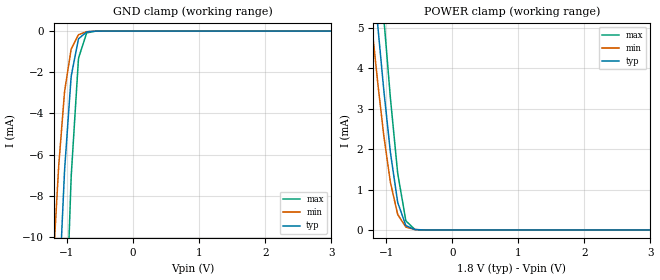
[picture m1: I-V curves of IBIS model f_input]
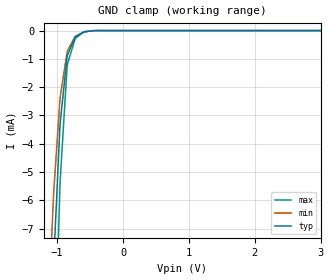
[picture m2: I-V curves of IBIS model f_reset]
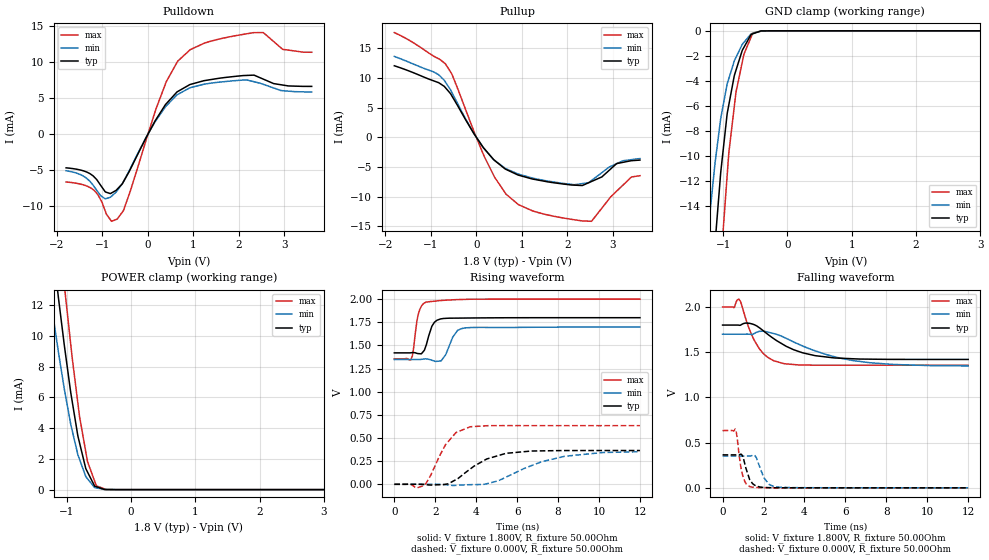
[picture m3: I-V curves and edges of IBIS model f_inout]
[IBIS Ver]   3.2
[File Name]   rc_p30_18v_64m_b.ibs
[File Rev]   1.01
[Date]   3/10/2010
[Source]   From silicon level SPICE model at Numonyx B.V.
[Notes]   The following information corresponds to the 65nm
   Redcliff P30 64Mb chip with EZBGA package.
[Disclaimer]   This information is for modeling purposes only and is not
   guaranteed.Numonyx B.V. is not responsible for any problem
   this model may cause to customers.
[Copyright]   Copyright 2010, Numonyx B.V., All Rights Reserved.
[Component]   P30_18V_64M_EZBGA
[Manufacturer]  Numonyx B.V.
[Package]
|   typ   min   max
R_pkg   0.35Ohm   0.18Ohm   0.51Ohm
L_pkg   7.00nH   3.67nH   10.32nH
C_pkg   1.26pF   0.74pF   1.77pF
[PIN]   signal_name   model_name   R_pin   L_pin   C_pin
A1   A1   f_input   0.29   6.04nH   1.07pF
A2   A6   f_input   0.38   7.66nH   1.33pF
A3   A8   f_input   0.23   4.81nH   0.86pF
A4   NC   NC
A5   A13   f_input   0.23   4.78nH   0.86pF
A6   VCC   POWER
A7   A18   f_input   0.30   6.53nH   1.17pF
A8   A22   f_input   0.35   7.76nH   1.27pF
B1   A2   f_input   0.29   5.78nH   1.02pF
B2   VSS   GND
B3   A9   f_input   0.36   7.42nH   1.29pF
B4   CE#   f_input   0.41   7.76nH   1.27pF
B5   A14   f_input   0.24   4.84nH   0.86pF
B6   NC   NC
B7   A19   f_input   0.29   6.32nH   1.13pF
B8   NC   NC
C1   A3   f_input   0.30   6.01nH   1.05pF
C2   A7   f_input   0.31   6.07nH   1.06pF
C3   A10   f_input   0.35   7.09nH   1.24pF
C4   A12   f_input   0.34   6.90nH   1.20pF
C5   A15   f_input   0.28   5.58nH   0.98pF
C6   WP#   f_input   0.28   5.60nH   0.99pF
C7   A20   f_input   0.43   8.80nH   1.52pF
C8   A21   f_input   0.35   7.07nH   1.24pF
D1   A4   f_input   0.32   6.32nH   1.10pF
D2   A5   f_input   0.30   5.77nH   1.00pF
D3   A11   f_input   0.37   7.56nH   1.31pF
D4   RST#   f_reset   0.35   6.65nH   1.20pF
D5   VCCQ   POWER
D6   VCCQ   POWER
D7   A16   f_input   0.28   5.43nH   0.94pF
D8   A17   f_input   0.30   5.95nH   1.04pF
E1   DQ8   f_inout   0.30   6.55nH   1.21pF
E2   DQ1   f_inout   0.28   5.48nH   1.04pF
E3   DQ9   f_inout   0.29   5.73nH   1.05pF
E4   DQ3   f_inout   0.26   5.08nH   0.96pF
E5   DQ4   f_inout   0.30   5.92nH   1.03pF
E6   CLK   f_input   0.30   5.91nH   1.12pF
E7   DQ15   f_inout   0.27   5.35nH   0.94pF
E8   NC   NC
F1   NC   NC
F2   DQ0   f_inout   0.22   4.43nH   0.86pF
F3   DQ10   f_inout   0.24   4.77nH   0.93pF
F4   DQ11   f_inout   0.24   4.76nH   0.92pF
F5   DQ12   f_inout   0.21   4.20nH   0.83pF
F6   ADV#   f_input   0.26   5.10nH   0.90pF
F7   WAIT   f_inout   0.24   4.85nH   0.92pF
F8   OE#   f_input   0.40   9.31nH   1.66pF
G1   A23   f_input   0.48   10.25nH   1.67pF
G2   NC   NC
G3   DQ2   f_inout   0.23   4.56nH   0.81pF
G4   NC   NC
G5   DQ5   f_inout   0.18   3.67nH   0.74pF
G6   DQ6   f_inout   0.19   3.89nH   0.79pF
G7   DQ14   f_inout   0.24   4.89nH   0.87pF
G8   WE#   f_input   0.51   10.32nH   1.77pF
H1   NC   NC
H2   VSS   GND
H3   NC   NC
H4   VSS   GND
H5   DQ13   f_inout   0.21   4.46nH   0.80pF
H6   VSS   GND
H7   DQ7   f_inout   0.25   5.06nH   0.90pF
H8   NC   NC
| Models and submodels in the file (3): f_input (Input), f_reset (Input), f_inout (I/O)
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[Model]   f_input
Model_type   Input
Vinl = 0.400V
Vinh = 1.400V
|   typ   min   max
C_comp   6.000pF   2.000pF   7.000pF
[Voltage Range]   1.800V   1.650V   2.000V
[Temperature Range]   25.0   85.0   -40.0
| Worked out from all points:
|   GND clamp passes 1 mA (typ) near -0.86 V on its own axis
|   POWER clamp passes 1 mA (typ) near -0.85 V on its own axis
[GND Clamp]
|   Voltage   I(typ)   I(min)   I(max)
-1.8V     -80.25mA   -59.1mA    -114.4mA
-1.206V   -19.7mA    -11.07mA   -35.87mA
-1.152V   -15.16mA   -8.009mA   -29.37mA
-1.125V   -12.92mA   -6.504mA   -26.13mA
-1.093V   -10.64mA   -5.183mA   -22.51mA
-1.033V   -6.563mA   -2.845mA   -15.96mA
-941.4mV  -2.368mA   -948.8uA   -7.426mA
-828mV    -400.8uA   -185.4uA   -1.397mA
-822.6mV  -364.5uA   -170.8uA   -1.276mA
-703.8mV  -43.48uA   -28.19uA   -98.9uA
-563.4mV  -3.074uA   -3.137uA   -3.274uA
3.6V      0A         0A         0A
[POWER Clamp]
|   Voltage   I(typ)   I(min)   I(max)
-1.8V     18.62mA    15.61mA    22.69mA
-1.211V   6.614mA    4.953mA    9.03mA
-1.12V    4.91mA     3.515mA    7.014mA
-1.033V   3.407mA    2.296mA    5.183mA
-963mV    2.323mA    1.48mA     3.786mA
-936mV    1.913mA    1.174mA    3.253mA
-828mV    699.7uA    395.3uA    1.428mA
-703.8mV  114.3uA    73.89uA    237.3uA
-698.4mV  105.3uA    68.73uA    218.4uA
-563.4mV  8.8uA      8.53uA     10.09uA
-412.2mV  495.2nA    779.4nA    260.9nA
3.6V      0A         0A         0A
[Model]   f_reset
Model_type   Input
Vinl = 0.400V
Vinh = 1.400V
|   typ   min   max
C_comp   6.000pF   2.000pF   7.000pF
[Voltage Range]   1.800V   1.650V   2.000V
[Temperature Range]   25.0   85.0   -40.0
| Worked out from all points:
|   GND clamp passes 1 mA (typ) near -0.85 V on its own axis
[GND Clamp]
|   Voltage   I(typ)   I(min)   I(max)
-1.8V     -77.85mA   -63.03mA   -101.5mA
-1.082V   -10.18mA   -7.202mA   -15.83mA
-1.076V   -9.791mA   -6.917mA   -15.29mA
-1.055V   -8.25mA    -5.779mA   -13.12mA
-1.033V   -7.154mA   -5.025mA   -11.41mA
-957.6mV  -3.346mA   -2.413mA   -5.432mA
-849.6mV  -921uA     -755.5uA   -1.269mA
-844.2mV  -866uA     -715.3uA   -1.181mA
-725.4mV  -224.5uA   -199.1uA   -275.8uA
-590.4mV  -43.29uA   -42.97uA   -41.36uA
-439.2mV  -1.59uA    -3.053uA   -485.9nA
3.6V      0A         0A         0A
[POWER Clamp]
|   Voltage   I(typ)   I(min)   I(max)
-1.8V     0A         0A         0A
0V        0A         0A         0A
1.651V    0A         0A         0A
1.802V    0A         0A         0A
2.002V    0A         0A         0A
3.6V      0A         0A         0A
[Model]   f_inout
Model_type   I/O
Vinl = 400.000mV
Vinh = 1.400V
Vmeas = 900.000mV
Cref = 30.000pF
|   typ   min   max
C_comp   4.000pF   2.000pF   5.000pF
[Voltage Range]   1.800V   1.700V   2.000V
[Temperature Range]   25.0   85.0   -40.0
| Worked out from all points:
|   slope of the pulldown table from 0 to 0.27 V, typ, clamps not added: 90.6 ohm
|   slope of the pullup table from 0 to 0.27 V, typ, clamps not added: 96.7 ohm
|   GND clamp passes 1 mA (typ) near -0.64 V on its own axis
|   POWER clamp passes 1 mA (typ) near -0.66 V on its own axis
|   falling waveform, V_fixture 1.800V, R_fixture 50.00Ohm: 20-80 % time 1.81ns typ, 2.79ns min, 867ps max; typ from 1.8 V to 1.42 V
|   rising waveform, V_fixture 1.800V, R_fixture 50.00Ohm: 20-80 % time 338ps typ, 439ps min, 268ps max; typ from 1.42 V to 1.8 V
|   rising waveform, V_fixture 0.000V, R_fixture 50.00Ohm: 20-80 % time 1.63ns typ, 2.53ns min, 970ps max; typ from 0.001 V to 0.365 V
|   falling waveform, V_fixture 0.000V, R_fixture 50.00Ohm: 20-80 % time 327ps typ, 428ps min, 259ps max; typ from 0.365 V to 0.001 V
[Pulldown]
|   Voltage   I(typ)   I(min)   I(max)
-1.8V     -4.722mA   -5.128mA   -6.695mA
-1.184V   -5.984mA   -7.328mA   -7.858mA
-941.4mV  -8.049mA   -9.026mA   -10.71mA
-801mV    -8.225mA   -8.679mA   -12.18mA
-676.8mV  -7.7mA     -7.894mA   -11.87mA
-536.4mV  -6.637mA   -6.606mA   -10.64mA
403.2mV   4.226mA    3.922mA    7.301mA
932.4mV   6.909mA    6.459mA    11.77mA
2.158V    8.16mA     7.549mA    13.96mA
2.531V    7.662mA    6.934mA    14.14mA
2.963V    6.824mA    6.038mA    11.8mA
3.6V      6.635mA    5.847mA    11.39mA
[GND Clamp]
|   Voltage   I(typ)   I(min)   I(max)
-1.8V     -76.26mA   -55.16mA   -98.01mA
-1.255V   -26.87mA   -17.37mA   -39.44mA
-1.211V   -23.37mA   -14.88mA   -35.12mA
-1.103V   -15.51mA   -9.625mA   -24.69mA
-1.012V   -10.06mA   -6.264mA   -16.72mA
-936mV    -6.559mA   -4.211mA   -11.41mA
-909mV    -5.821mA   -3.762mA   -9.605mA
-801mV    -3.151mA   -2.12mA    -4.911mA
-676.8mV  -1.316mA   -920.1uA   -1.86mA
-563.4mV  -281.3uA   -234.6uA   -473.7uA
-385.2mV  -6.376uA   -10.08uA   -1.133uA
3.6V      0A         0A         0A
[Pullup]
|   Voltage   I(typ)   I(min)   I(max)
-1.8V     12.03mA    13.6mA     17.61mA
-936mV    9.49mA     10.99mA    13.65mA
-676.8mV  8.335mA    9.289mA    12.35mA
-536.4mV  6.975mA    7.559mA    10.64mA
-50.4mV   613.4uA    628uA      996.6uA
403.2mV   -3.891mA   -3.876mA   -6.696mA
932.4mV   -6.379mA   -6.207mA   -11.35mA
2.158V    -8.051mA   -7.978mA   -13.88mA
2.536V    -7.434mA   -7.273mA   -14.13mA
3.087V    -4.431mA   -4.44mA    -9.072mA
3.416V    -3.938mA   -3.759mA   -6.674mA
3.6V      -3.841mA   -3.589mA   -6.464mA
[POWER Clamp]
|   Voltage   I(typ)   I(min)   I(max)
-1.8V     38.66mA    30.29mA    47.7mA
-1.255V   17.06mA    12.59mA    22.58mA
-1.13V    12.57mA    9.011mA    17.23mA
-1.017V   8.787mA    6.092mA    12.54mA
-936mV    6.295mA    4.237mA    9.423mA
-801mV    3.059mA    1.98mA     4.786mA
-703.8mV  1.383mA    855.8uA    2.475mA
-676.8mV  1.148mA    708.4uA    1.834mA
-563.4mV  220uA      130.1uA    529uA
-536.4mV  182.2uA    107.9uA    244.5uA
-385.2mV  6.239uA    4.464uA    4.885uA
3.6V      0A         0A         0A
[Ramp]
R_load = 50.00Ohm
|   typ   min   max
dV/dt_r   218.602mV/1.625ns   210.755mV/2.530ns   379.823mV/969.838ps
dV/dt_f   227.872mV/1.814ns   210.690mV/2.790ns   386.231mV/866.778ps
[Falling Waveform]
V_fixture = 1.800V
V_fixture_min = 1.700V
V_fixture_max = 2.000V
R_fixture = 50.00Ohm
|   Time   V(typ)   V(min)   V(max)
0s        1.799V     1.698V     1.999V
560ps     1.799V     1.698V     1.992V
800ps     1.797V     1.698V     2.085V
1.34ns    1.817V     1.697V     1.735V
1.79ns    1.77V      1.729V     1.54V
2.19ns    1.7V       1.722V     1.445V
3.01ns    1.577V     1.662V     1.372V
4.51ns    1.461V     1.515V     1.356V
6.37ns    1.427V     1.407V     1.355V
12ns      1.419V     1.347V     1.355V
[Rising Waveform]
V_fixture = 1.800V
V_fixture_min = 1.700V
V_fixture_max = 2.000V
R_fixture = 50.00Ohm
|   Time   V(typ)   V(min)   V(max)
0s        1.419V     1.347V     1.355V
800ps     1.42V      1.347V     1.344V
880ps     1.422V     1.347V     1.386V
1.17ns    1.411V     1.347V     1.836V
1.55ns    1.499V     1.354V     1.967V
2.08ns    1.771V     1.328V     1.98V
2.51ns    1.792V     1.4V       1.988V
3.09ns    1.794V     1.661V     1.994V
3.46ns    1.795V     1.688V     1.996V
12ns      1.799V     1.698V     1.999V
[Rising Waveform]
V_fixture = 0.000V
V_fixture_min = 0.000V
V_fixture_max = 0.000V
R_fixture = 50.00Ohm
|   Time   V(typ)   V(min)   V(max)
0s        808.8uV    974.4uV    564.8uV
1.43ns    -1.175mV   610.6uV    -12.94mV
1.78ns    -7.224mV   1.984mV    99.04mV
2.5ns     1.328mV    -3.965mV   427.7mV
3.01ns    50.96mV    -10.88mV   558.7mV
3.71ns    166mV      -3.447mV   621.7mV
4.51ns    273.4mV    6.371mV    632.6mV
5.46ns    335mV      78.32mV    634.1mV
8.33ns    364.7mV    303.2mV    633.7mV
12ns      365.1mV    352.2mV    633.6mV
[Falling Waveform]
V_fixture = 0.000V
V_fixture_min = 0.000V
V_fixture_max = 0.000V
R_fixture = 50.00Ohm
|   Time   V(typ)   V(min)   V(max)
0s        365.1mV    352.2mV    633.6mV
630ps     365.2mV    352.2mV    645.2mV
880ps     371.9mV    352.2mV    246.2mV
1.01ns    329.3mV    352.3mV    113.9mV
1.43ns    58.72mV    356.5mV    9.022mV
1.65ns    21.41mV    334.2mV    5.102mV
2.01ns    4.999mV    115mV      2.94mV
2.28ns    2.436mV    37.75mV    2.11mV
2.68ns    1.655mV    10.26mV    1.362mV
12ns      808.8uV    974.4uV    564.8uV
